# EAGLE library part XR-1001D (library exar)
General purpose low pass FILTER
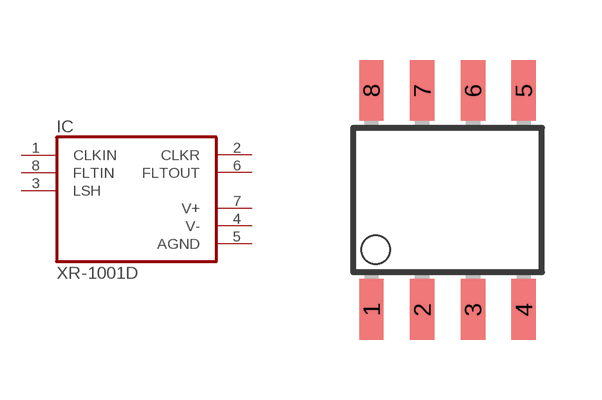
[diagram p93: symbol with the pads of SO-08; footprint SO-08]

Designator prefix IC

## XR-1001D (OC_FARNELL: unknown; OC_NEWARK: unknown)  [SO-08]
1  CLKIN  in
2  CLKR  out
3  LSH  in
4  V-  pwr
5  AGND  pwr
6  FLTOUT  out
7  V+  pwr
8  FLTIN  in

## Footprint SO-08 (pad centres in mm)
Small Outline Package
smd 0.61 x 1.524: 1 -1.27,-2.743; 2 0,-2.743; 3 1.27,-2.743; 4 2.54,-2.743; 5 2.54,2.743; 6 1.27,2.743; 7 0,2.743; 8 -1.27,2.743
